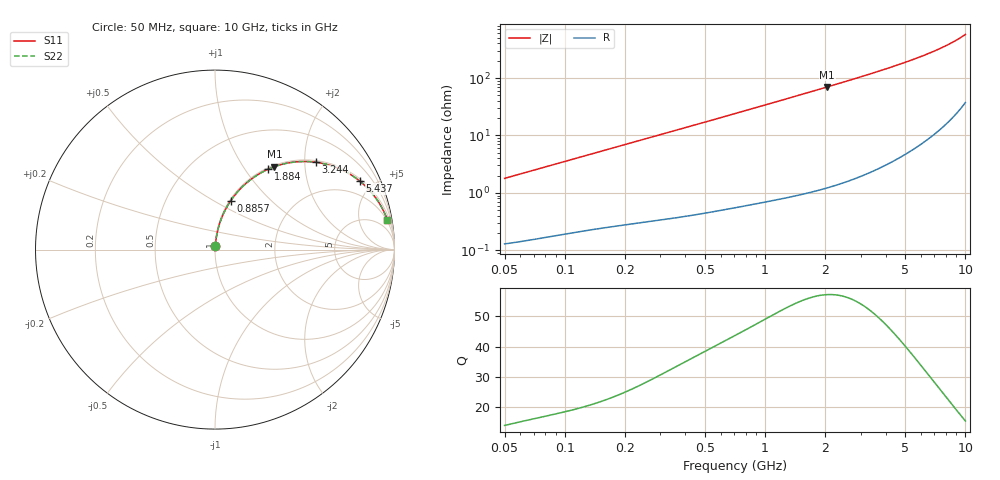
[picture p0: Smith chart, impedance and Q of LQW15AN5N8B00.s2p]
!Murata Part Number: LQW15AN5N8B00
!These Parameters are Measured in Series Mode Connection
!  o--[Z]--o
!Port1  Port2
!  o-------o
!Freq. Start=50[MHz] Stop=10[GHz], 401[Steps]
# Hz S RI R 50
!Freq.(Hz)	S 11(Real)	S 11(Imag)	S 21(Real)	S 21(Imag)	S 12(Real)	S 12(Imag)	S 22(Real)	S 22(Imag)
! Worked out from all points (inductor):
!   401 points, 50 MHz to 10 GHz, reference 50 ohm
!   read as one part in series: L = 5.65 nH near 51.34 MHz
!   highest Q = 57.2 at 2.04 GHz (marker M1), where L = 5.45 nH
!   S11 on the Smith chart (normalised r, x): 50 MHz: 1.00, +0.04; 885.7 MHz: 1.01, +0.60; 1.884 GHz: 1.02, +1.29; 3.244 GHz: 1.04, +2.28; 5.437 GHz: 1.11, +4.16; 10 GHz: 2, +11
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5e7  0.00161 0.0178  0.9984 -0.0178  0.9984 -0.0178  0.00161 0.0178
1.214486e8  0.00393 0.0422  0.9961 -0.0422  0.9961 -0.0422  0.00393 0.0422
1.956524e8  0.00725 0.0669  0.9928 -0.0669  0.9928 -0.0669  0.00725 0.0669
2.949953e8  0.0134 0.0995  0.9866 -0.0995  0.9866 -0.0995  0.0134 0.0995
4.628099e8  0.0282 0.1527  0.9718 -0.1527  0.9718 -0.1527  0.0282 0.1527
7.071068e8  0.0592 0.2248  0.9408 -0.2248  0.9408 -0.2248  0.0592 0.2248
8.85684e8  0.0877 0.2725  0.9123 -0.2725  0.9123 -0.2725  0.0877 0.2725
1.052113e9  0.1179 0.3127  0.8821 -0.3127  0.8821 -0.3127  0.1179 0.3127
1.249815e9  0.1573 0.3547  0.8427 -0.3547  0.8427 -0.3547  0.1573 0.3547
1.465132e9  0.2031 0.3933  0.7969 -0.3933  0.7969 -0.3933  0.2031 0.3933
1.717543e9  0.259 0.4293  0.741 -0.4293  0.741 -0.4293  0.259 0.4293
1.884411e9  0.2962 0.4479  0.7038 -0.4479  0.7038 -0.4479  0.2962 0.4479
2.040286e9  0.3306 0.4618  0.6694 -0.4618  0.6694 -0.4618  0.3306 0.4618
2.589628e9  0.4459 0.4883  0.5541 -0.4883  0.5541 -0.4883  0.4459 0.4883
3.243629e9  0.5637 0.4865  0.4363 -0.4865  0.4363 -0.4865  0.5637 0.4865
3.654301e9  0.6256 0.474  0.3744 -0.474  0.3744 -0.474  0.6256 0.474
4.171863e9  0.6913 0.4512  0.3087 -0.4512  0.3087 -0.4512  0.6913 0.4512
5.437278e9  0.8059 0.3823  0.1941 -0.3823  0.1941 -0.3823  0.8059 0.3823
6.458996e9  0.8652 0.3258  0.1348 -0.3258  0.1348 -0.3258  0.8652 0.3258
7.571744e9  0.9086 0.2691  0.0914 -0.2691  0.0914 -0.2691  0.9086 0.2691
8.644138e9  0.9368 0.2201  0.0632 -0.2201  0.0632 -0.2201  0.9368 0.2201
1e10  0.9603 0.1653  0.0397 -0.1653  0.0397 -0.1653  0.9603 0.1653
